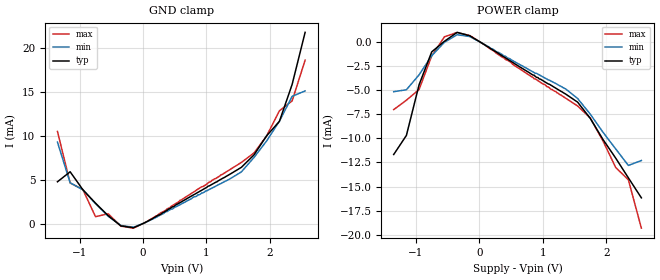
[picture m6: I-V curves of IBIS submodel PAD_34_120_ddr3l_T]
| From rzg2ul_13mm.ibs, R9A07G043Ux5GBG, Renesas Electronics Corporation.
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[Submodel]  PAD_34_120_ddr3l_T
Submodel_type Dynamic_clamp
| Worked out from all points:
|   GND clamp passes 1 mA (typ) near -0.57 V on its own axis
[GND Clamp]
| Voltage   I(typ)   I(min)   I(max)
-1.35V    4.75mA     9.26mA     10.48mA
-1.15V    5.89mA     4.64mA     4.616mA
-950mV    3.853mA    3.837mA    3.872mA
-750mV    2.319mA    2.27mA     781uA
-550mV    892.6uA    836.8uA    1.11mA
-350mV    -268.3uA   -216.8uA   -298.6uA
-150mV    -477.7uA   -416.8uA   -522.4uA
1.36V     5.57mA     5.045mA    6.094mA
1.75V     7.818mA    7.529mA    8.036mA
2.15V     11.63mA    11.64mA    12.83mA
2.35V     15.82mA    14.47mA    13.95mA
2.555V    21.75mA    15.09mA    18.59mA
[POWER Clamp]
| Voltage   I(typ)   I(min)   I(max)
-1.35V    -11.68mA   -5.186mA   -7.039mA
-1.15V    -9.711mA   -4.988mA   -6.067mA
-950mV    -4.476mA   -3.447mA   -4.96mA
-750mV    -1.067mA   -1.467mA   -1.479mA
-550mV    23.63uA    -78.87uA   489.3uA
-350mV    944uA      700.5uA    935.6uA
-150mV    585.2uA    510.8uA    617.1uA
1.36V     -5.427mA   -4.893mA   -5.853mA
1.75V     -7.951mA   -7.516mA   -7.918mA
2.15V     -12.05mA   -11.1mA    -13.02mA
2.35V     -14.09mA   -12.81mA   -14.29mA
2.555V    -16.16mA   -12.3mA    -19.29mA
